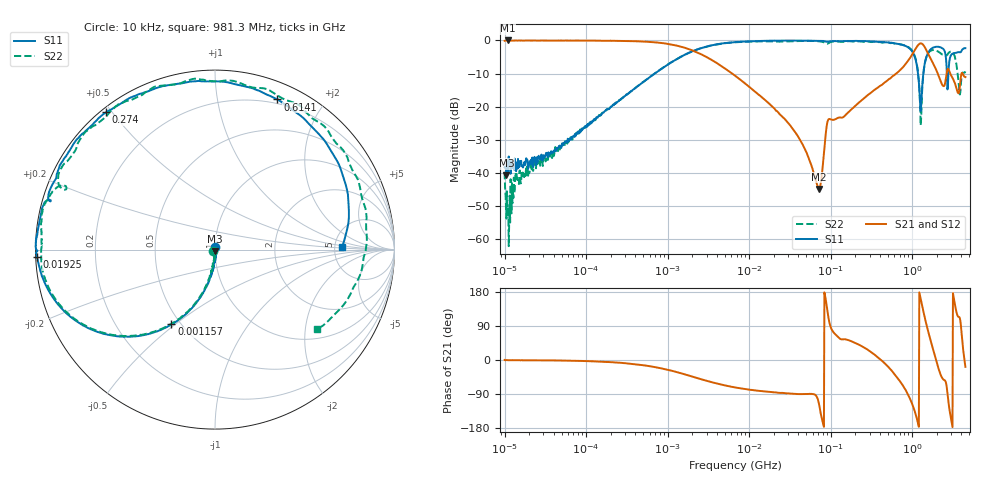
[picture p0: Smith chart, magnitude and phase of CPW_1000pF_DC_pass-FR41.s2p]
!Siglent Technologies,SNA5004A,SNA5XCED5R0097,V1.0.0.2.10.R9
!Date: 2024-10-29 18:17:33
!Data & Calibration Information:
!Freq	S11:F2(ON)	S21:F2(ON)	S12:F2(ON)	S22:F2(ON)
# Hz S DB R 50
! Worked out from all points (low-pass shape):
!   1001 points, 10 kHz to 4.5 GHz, reference 50 ohm
!   highest |S21| = 0.00 dB at 10.95 kHz (marker M1); lowest = -44.9 dB at 71.7 MHz (marker M2)
!   |S21| within 3 dB of the highest: start of sweep to 2.008 MHz; 1.071 GHz to 1.499 GHz (428.7 MHz wide, 33.4 % of centre)
!   lowest |S11| = -40.7 dB at 10.53 kHz (marker M3), VSWR 1.02, Z = 49.9 - j0.91 ohm
!   |S11| at or under -10 dB: start of sweep to 694.1 kHz; 1.18 GHz to 1.371 GHz (190.6 MHz wide, 14.9 % of centre); 2.667 GHz to 2.784 GHz (117.8 MHz wide, 4.32 % of centre)
!   |S22| runs from -62.1 to -0.1 dB; largest |S21 - S12| = 0.0086
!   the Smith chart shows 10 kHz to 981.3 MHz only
!   S11 on the Smith chart (normalised r, x): 10 kHz: 1.00, +0.02; 1.157 MHz: 0.45, -0.48; 19.25 MHz: 0.00, -0.02; 274 MHz: 0.01, +0.48; 614.1 MHz: 0.16, +1.49; 981.3 MHz: 5.84, +0.35
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10000  -38.30 86.6  -0.10 0.0  -0.03 -0.0  -39.76 -147.2
10534.47  -40.75 -96.5  -0.05 -0.1  -0.01 -0.5  -53.78 113.4
10953.99  -39.69 -73.6  -0.00 -0.6  0.02 -0.5  -50.87 -47.1
87919.76  -27.25 -88.3  -0.04 -2.5  -0.01 -2.7  -26.96 -92.5
772988.4  -9.17 -111.4  -0.67 -20.6  -0.64 -20.7  -9.16 -112.0
1157238  -6.35 -120.2  -1.31 -29.1  -1.28 -29.3  -6.33 -120.7
6708204  -0.50 -164.0  -10.63 -72.4  -10.60 -72.6  -0.55 -164.4
1.92538e7  -0.08 -177.6  -19.98 -84.8  -19.94 -85.1  -0.28 -178.7
5.897837e7  -0.09 170.0  -38.24 -89.3  -38.12 -89.8  -0.15 166.0
7.169534e7  -0.08 166.8  -44.85 -114.5  -44.76 -114.3  -0.28 162.0
9.546883e7  -0.33 163.6  -23.73 103.4  -23.68 103.5  -0.75 158.3
2.740134e8  -0.21 128.4  -16.85 29.3  -16.79 29.2  -0.33 112.3
5.185364e8  -0.61 84.4  -11.68 -20.1  -11.64 -20.0  -0.63 58.9
6.141451e8  -0.86 67.4  -10.30 -38.4  -10.21 -38.4  -0.89 39.4
9.812658e8  -2.99 1.2  -4.61 -111.4  -4.50 -111.2  -2.84 -38.1
1.431297e9  -6.80 37.7  -2.07 110.9  -2.03 111.1  -6.93 3.2
1.762711e9  -2.31 -21.3  -6.44 36.2  -6.38 36.4  -2.95 -89.5
2.115077e9  -1.94 -73.7  -10.74 -23.9  -10.67 -23.5  -3.48 -177.0
2.638948e9  -7.53 148.2  -10.26 -66.9  -10.17 -66.6  -4.59 78.3
3.20796e9  -3.93 175.7  -11.82 169.1  -11.73 169.6  -3.82 -26.1
3.750313e9  -3.53 76.2  -15.71 113.5  -15.68 113.9  -13.74 -161.2
4.5e9  -2.32 -33.5  -11.05 -18.1  -11.06 -18.9  -9.35 -178.6
